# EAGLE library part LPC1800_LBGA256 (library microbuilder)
Generic LPC1800 LBGA256 Package
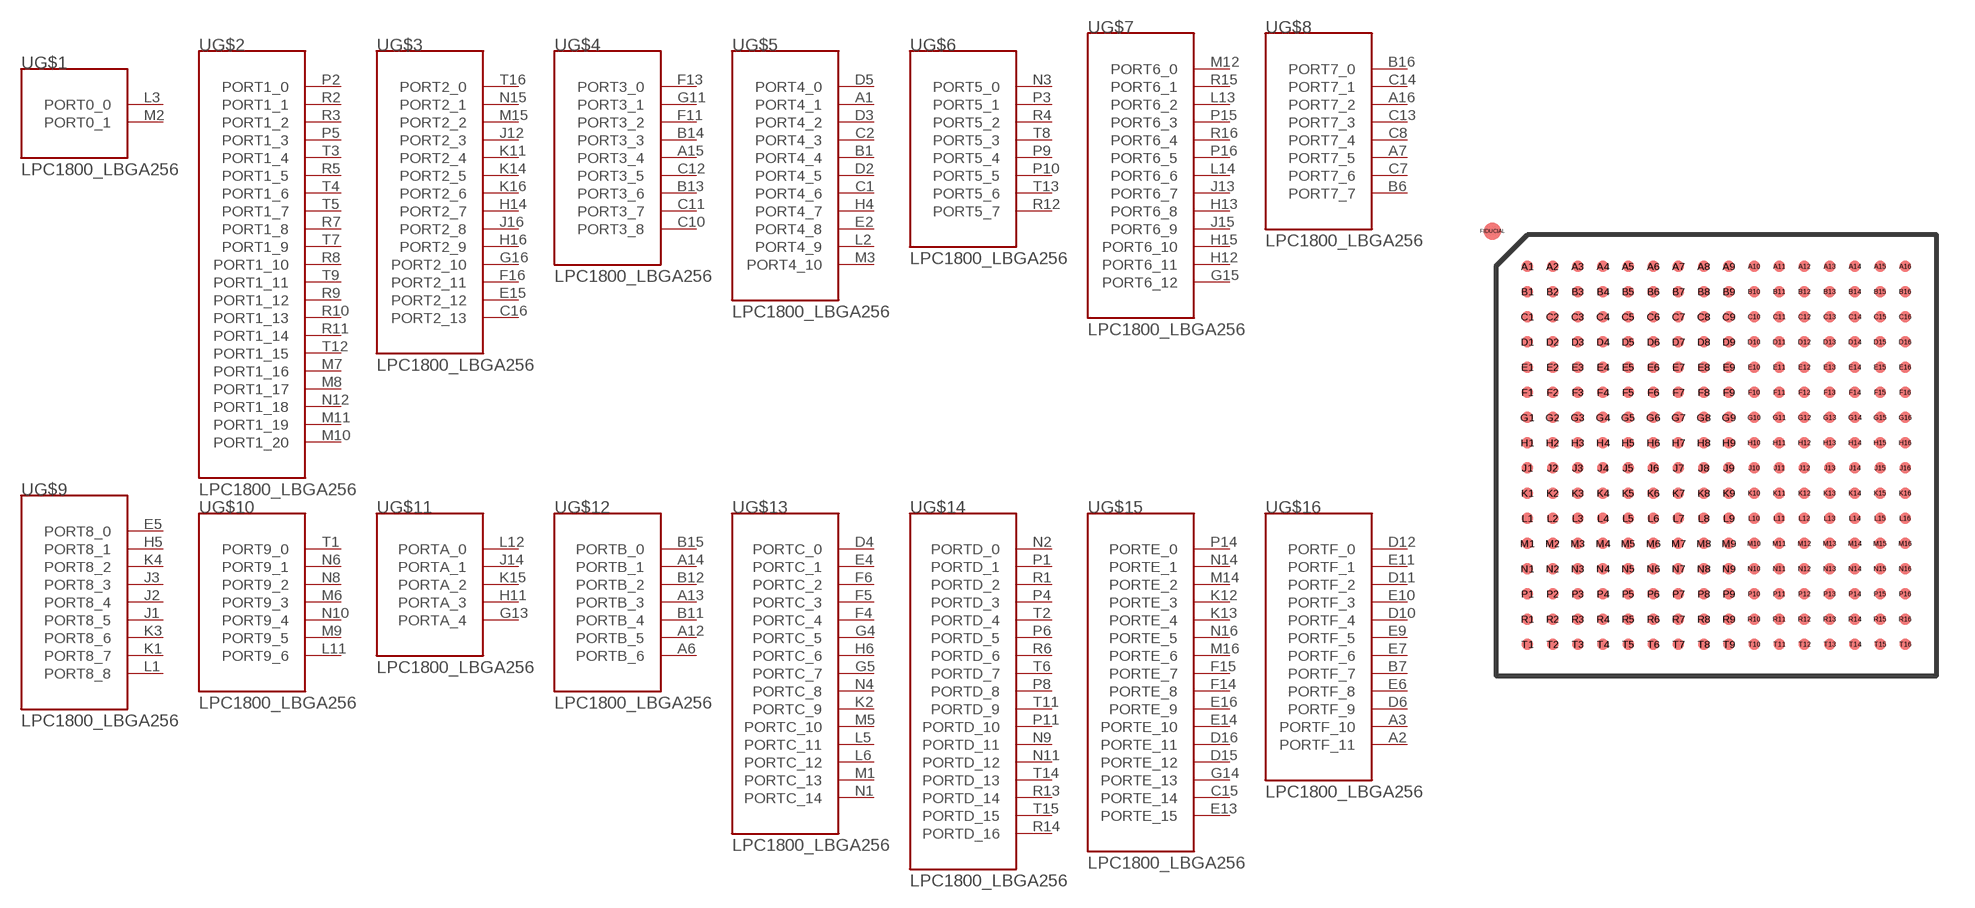
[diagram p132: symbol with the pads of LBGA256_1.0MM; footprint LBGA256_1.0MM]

Designator prefix U; gates G$1=LPC1800_PORT0 G$2=LPC1800_PORT1 G$3=LPC1800_PORT2 G$4=LPC1800_PORT3 G$5=LPC1800_PORT4 G$6=LPC1800_PORT5 G$7=LPC1800_PORT6 G$8=LPC1800_PORT7 G$9=LPC1800_PORT8 G$10=LPC1800_PORT9 G$11=LPC1800_PORTA G$12=LPC1800_PORTB G$13=LPC1800_PORTC G$14=LPC1800_PORTD G$15=LPC1800_PORTE G$16=LPC1800_PORTF G$17=LPC1800_ANA G$18=LPC1800_AO G$19=LPC1800_CLK G$20=LPC1800_DBUG G$21=LPC1800_SUP G$22=LPC1800_USB G$23=LPC1800_I2C

## LPC1800_LBGA256  [LBGA256_1.0MM]
A1  G$5:PORT4_1
A2  G$16:PORTF_11
A3  G$16:PORTF_10
A4  G$17:ADC2
A5  G$17:ADC6
A6  G$12:PORTB_6
A7  G$8:PORT7_5
A8  G$18:RTCX1
A9  G$18:WAKEUP0
A10  G$18:WAKEUP1
A11  G$18:ALARM
A12  G$12:PORTB_5
A13  G$12:PORTB_3
A14  G$12:PORTB_1
A15  G$4:PORT3_4
A16  G$8:PORT7_2
B1  G$5:PORT4_4
B2  G$17:VSSA  sup
B3  G$17:ADC5
B4  G$17:VDDA  sup
B5  G$17:ADC3
B6  G$8:PORT7_7
B7  G$16:PORTF_7
B8  G$18:RTXC2
B9  G$18:SAMPLE_N
B10  G$18:VBAT
B11  G$12:PORTB_4
B12  G$12:PORTB_2
B13  G$4:PORT3_6
B14  G$4:PORT3_3
B15  G$12:PORTB_0
B16  G$8:PORT7_0
C1  G$5:PORT4_6
C2  G$5:PORT4_3
C3  G$17:ADC1
C4  G$21:VSS  sup
C5  G$17:ADC7
C6  G$17:ADC4
C7  G$8:PORT7_6
C8  G$8:PORT7_4
C9  G$18:WAKEUP2
C10  G$4:PORT3_8
C11  G$4:PORT3_7
C12  G$4:PORT3_5
C13  G$8:PORT7_3
C14  G$8:PORT7_1
C15  G$15:PORTE_14
C16  G$3:PORT2_13
D1  G$19:XTAL1
D2  G$5:PORT4_5
D3  G$5:PORT4_2
D4  G$13:PORTC_0
D5  G$5:PORT4_0
D6  G$16:PORTF_9
D7  G$21:VDDE  sup
D8  G$18:WAKEUP3
D9  G$18:RESET
D10  G$16:PORTF_4
D11  G$16:PORTF_2
D12  G$16:PORTF_0
D13  G$21:VSS  sup
D14  G$19:CLK2
D15  G$15:PORTE_12
D16  G$15:PORTE_11
E1  G$19:XTAL2
E2  G$5:PORT4_8
E3  G$17:ADC0
E4  G$13:PORTC_1
E5  G$9:PORT8_0
E6  G$16:PORTF_8
E7  G$16:PORTF_6
E8  G$21:VPP  sup
E9  G$16:PORTF_5
E10  G$16:PORTF_3
E11  G$16:PORTF_1
E12  G$21:VDDE  sup
E13  G$15:PORTE_15
E14  G$15:PORTE_10
E15  G$3:PORT2_12
E16  G$15:PORTE_9
F1  G$22:USB_VBUS
F2  G$22:USB_DP0
F3  G$22:USB_VDDA3V3_DRIVER
F4  G$13:PORTC_4
F5  G$13:PORTC_3
F6  G$13:PORTC_2
F7  G$21:VDDE  sup
F8  G$21:VDDE  sup
F9  G$21:VDDC  sup
F10  G$21:VDDC  sup
F11  G$4:PORT3_2
F12  G$22:USB_DP1
F13  G$4:PORT3_0
F14  G$15:PORTE_8
F15  G$15:PORTE_7
F16  G$3:PORT2_11
G1  G$22:USB_VSSA_REF
G2  G$22:USB_DM0
G3  G$22:USB_VDDA3V3
G4  G$13:PORTC_5
G5  G$13:PORTC_7
G6  G$21:VSS  sup
G7  G$21:VSS  sup
G8  G$21:VSS  sup
G9  G$21:VSS  sup
G10  G$21:VDDE  sup
G11  G$4:PORT3_1
G12  G$22:USB_DM1
G13  G$11:PORTA_4
G14  G$15:PORTE_13
G15  G$7:PORT6_12
G16  G$3:PORT2_10
H1  G$22:USB_RREF
H2  G$22:USB_ID
H3  G$22:USB_VSSA_TERM
H4  G$5:PORT4_7
H5  G$9:PORT8_1
H6  G$13:PORTC_6
H7  G$21:VSS  sup
H8  G$21:VSS  sup
H9  G$21:VSS  sup
H10  G$21:VDDE  sup
H11  G$11:PORTA_3
H12  G$7:PORT6_11
H13  G$7:PORT6_8
H14  G$3:PORT2_7
H15  G$7:PORT6_10
H16  G$3:PORT2_9
J1  G$9:PORT8_5
J2  G$9:PORT8_4
J3  G$9:PORT8_3
J4  G$20:TDI
J5  G$20:TCK
J6  G$21:VDDE  sup
J7  G$21:VDDE  sup
J8  G$21:VSS  sup
J9  G$21:VSS  sup
J10  G$21:VSS  sup
J11  G$21:VSS  sup
J12  G$3:PORT2_3
J13  G$7:PORT6_7
J14  G$11:PORTA_1
J15  G$7:PORT6_9
J16  G$3:PORT2_8
K1  G$9:PORT8_7
K2  G$13:PORTC_9
K3  G$9:PORT8_6
K4  G$9:PORT8_2
K5  G$20:TDO
K6  G$20:TMS
K7  G$21:VDDE  sup
K8  G$21:VSS  sup
K9  G$21:VSS  sup
K10  G$21:VSS  sup
K11  G$3:PORT2_4
K12  G$15:PORTE_3
K13  G$15:PORTE_4
K14  G$3:PORT2_5
K15  G$11:PORTA_2
K16  G$3:PORT2_6
L1  G$9:PORT8_8  sup
L2  G$5:PORT4_9
L3  G$1:PORT0_0
L4  G$20:DBGEN
L5  G$13:PORTC_11
L6  G$13:PORTC_12
L7  G$21:VDDC  sup
L8  G$21:VDDC  sup
L9  G$21:VDDE  sup
L10  G$21:VDDE  sup
L11  G$10:PORT9_6
L12  G$11:PORTA_0
L13  G$7:PORT6_2
L14  G$7:PORT6_6
L15  G$23:SCL  sup
L16  G$23:SDA  sup
M1  G$13:PORTC_13
M2  G$1:PORT0_1
M3  G$5:PORT4_10
M4  G$20:TRST
M5  G$13:PORTC_10
M6  G$10:PORT9_3
M7  G$2:PORT1_16
M8  G$2:PORT1_17
M9  G$10:PORT9_5
M10  G$2:PORT1_20
M11  G$2:PORT1_19
M12  G$7:PORT6_0
M13  G$21:VSS  sup
M14  G$15:PORTE_2
M15  G$3:PORT2_2
M16  G$15:PORTE_6
N1  G$13:PORTC_14
N2  G$14:PORTD_0
N3  G$6:PORT5_0
N4  G$13:PORTC_8
N5  G$19:CLK0
N6  G$10:PORT9_1
N7  G$21:VDDE  sup
N8  G$10:PORT9_2
N9  G$14:PORTD_11
N10  G$10:PORT9_4
N11  G$14:PORTD_12
N12  G$2:PORT1_18
N13  G$21:VDDE  sup
N14  G$15:PORTE_1
N15  G$3:PORT2_1
N16  G$15:PORTE_5
P1  G$14:PORTD_1
P2  G$2:PORT1_0
P3  G$6:PORT5_1
P4  G$14:PORTD_3
P5  G$2:PORT1_3
P6  G$14:PORTD_5
P7  G$21:VSS  sup
P8  G$14:PORTD_8
P9  G$6:PORT5_4
P10  G$6:PORT5_5
P11  G$14:PORTD_10
P12  G$19:CLK3
P13  G$21:VSS  sup
P14  G$15:PORTE_0
P15  G$7:PORT6_3
P16  G$7:PORT6_5
R1  G$14:PORTD_2
R2  G$2:PORT1_1
R3  G$2:PORT1_2
R4  G$6:PORT5_2
R5  G$2:PORT1_5
R6  G$14:PORTD_6
R7  G$2:PORT1_8
R8  G$2:PORT1_10
R9  G$2:PORT1_12
R10  G$2:PORT1_13
R11  G$2:PORT1_14
R12  G$6:PORT5_7
R13  G$14:PORTD_14
R14  G$14:PORTD_16
R15  G$7:PORT6_1
R16  G$7:PORT6_4
T1  G$10:PORT9_0
T2  G$14:PORTD_4
T3  G$2:PORT1_4
T4  G$2:PORT1_6
T5  G$2:PORT1_7
T6  G$14:PORTD_7
T7  G$2:PORT1_9
T8  G$6:PORT5_3
T9  G$2:PORT1_11
T10  G$19:CLK1
T11  G$14:PORTD_9
T12  G$2:PORT1_15
T13  G$6:PORT5_6
T14  G$14:PORTD_13
T15  G$14:PORTD_15
T16  G$3:PORT2_0

## Footprint LBGA256_1.0MM (pad centres in mm)
LBGA256 - SOT740-2 LBGA256: plastic low profile ball grid array package; 256 balls; body 17 x 17 x 1 mm
smd 0.45 x 0.45: A1 -7.5,7.5; A2 -6.5,7.5; A3 -5.5,7.5; A4 -4.5,7.5; A5 -3.5,7.5; A6 -2.5,7.5; A7 -1.5,7.5; A8 -0.5,7.5; A9 0.5,7.5; A10 1.5,7.5; A11 2.5,7.5; A12 3.5,7.5; A13 4.5,7.5; A14 5.5,7.5; A15 6.5,7.5; A16 7.5,7.5; B1 -7.5,6.5; B2 -6.5,6.5; B3 -5.5,6.5; B4 -4.5,6.5; B5 -3.5,6.5; B6 -2.5,6.5; B7 -1.5,6.5; B8 -0.5,6.5; B9 0.5,6.5; B10 1.5,6.5; B11 2.5,6.5; B12 3.5,6.5; B13 4.5,6.5; B14 5.5,6.5; B15 6.5,6.5; B16 7.5,6.5; C1 -7.5,5.5; C2 -6.5,5.5; C3 -5.5,5.5; C4 -4.5,5.5; C5 -3.5,5.5; C6 -2.5,5.5; C7 -1.5,5.5; C8 -0.5,5.5; C9 0.5,5.5; C10 1.5,5.5; C11 2.5,5.5; C12 3.5,5.5; C13 4.5,5.5; C14 5.5,5.5; C15 6.5,5.5; C16 7.5,5.5; D1 -7.5,4.5; D2 -6.5,4.5; D3 -5.5,4.5; D4 -4.5,4.5; D5 -3.5,4.5; D6 -2.5,4.5; D7 -1.5,4.5; D8 -0.5,4.5; D9 0.5,4.5; D10 1.5,4.5; D11 2.5,4.5; D12 3.5,4.5; D13 4.5,4.5; D14 5.5,4.5; D15 6.5,4.5; D16 7.5,4.5; E1 -7.5,3.5; E2 -6.5,3.5; E3 -5.5,3.5; E4 -4.5,3.5; E5 -3.5,3.5; E6 -2.5,3.5; E7 -1.5,3.5; E8 -0.5,3.5; E9 0.5,3.5; E10 1.5,3.5; E11 2.5,3.5; E12 3.5,3.5; E13 4.5,3.5; E14 5.5,3.5; E15 6.5,3.5; E16 7.5,3.5; F1 -7.5,2.5; F2 -6.5,2.5; F3 -5.5,2.5; F4 -4.5,2.5; F5 -3.5,2.5; F6 -2.5,2.5; F7 -1.5,2.5; F8 -0.5,2.5; F9 0.5,2.5; F10 1.5,2.5; F11 2.5,2.5; F12 3.5,2.5; F13 4.5,2.5; F14 5.5,2.5; F15 6.5,2.5; F16 7.5,2.5; G1 -7.5,1.5; G2 -6.5,1.5; G3 -5.5,1.5; G4 -4.5,1.5; G5 -3.5,1.5; G6 -2.5,1.5; G7 -1.5,1.5; G8 -0.5,1.5; G9 0.5,1.5; G10 1.5,1.5; G11 2.5,1.5; G12 3.5,1.5; G13 4.5,1.5; G14 5.5,1.5; G15 6.5,1.5; G16 7.5,1.5; H1 -7.5,0.5; H2 -6.5,0.5; H3 -5.5,0.5; H4 -4.5,0.5; H5 -3.5,0.5; H6 -2.5,0.5; H7 -1.5,0.5; H8 -0.5,0.5; H9 0.5,0.5; H10 1.5,0.5; H11 2.5,0.5; H12 3.5,0.5; H13 4.5,0.5; H14 5.5,0.5; H15 6.5,0.5; H16 7.5,0.5; J1 -7.5,-0.5; J2 -6.5,-0.5; J3 -5.5,-0.5; J4 -4.5,-0.5; J5 -3.5,-0.5; J6 -2.5,-0.5; J7 -1.5,-0.5; J8 -0.5,-0.5; J9 0.5,-0.5; J10 1.5,-0.5; J11 2.5,-0.5; J12 3.5,-0.5; J13 4.5,-0.5; J14 5.5,-0.5; J15 6.5,-0.5; J16 7.5,-0.5; K1 -7.5,-1.5; K2 -6.5,-1.5; K3 -5.5,-1.5; K4 -4.5,-1.5; K5 -3.5,-1.5; K6 -2.5,-1.5; K7 -1.5,-1.5; K8 -0.5,-1.5; K9 0.5,-1.5; K10 1.5,-1.5; K11 2.5,-1.5; K12 3.5,-1.5; K13 4.5,-1.5; K14 5.5,-1.5; K15 6.5,-1.5; K16 7.5,-1.5; L1 -7.5,-2.5; L2 -6.5,-2.5; L3 -5.5,-2.5; L4 -4.5,-2.5; L5 -3.5,-2.5; L6 -2.5,-2.5; L7 -1.5,-2.5; L8 -0.5,-2.5; L9 0.5,-2.5; L10 1.5,-2.5; L11 2.5,-2.5; L12 3.5,-2.5; L13 4.5,-2.5; L14 5.5,-2.5; L15 6.5,-2.5; L16 7.5,-2.5; M1 -7.5,-3.5; M2 -6.5,-3.5; M3 -5.5,-3.5; M4 -4.5,-3.5; M5 -3.5,-3.5; M6 -2.5,-3.5; M7 -1.5,-3.5; M8 -0.5,-3.5; M9 0.5,-3.5; M10 1.5,-3.5; M11 2.5,-3.5; M12 3.5,-3.5; M13 4.5,-3.5; M14 5.5,-3.5; M15 6.5,-3.5; M16 7.5,-3.5; N1 -7.5,-4.5; N2 -6.5,-4.5; N3 -5.5,-4.5; N4 -4.5,-4.5; N5 -3.5,-4.5; N6 -2.5,-4.5; N7 -1.5,-4.5; N8 -0.5,-4.5; N9 0.5,-4.5; N10 1.5,-4.5; N11 2.5,-4.5; N12 3.5,-4.5; N13 4.5,-4.5; N14 5.5,-4.5; N15 6.5,-4.5; N16 7.5,-4.5; P1 -7.5,-5.5; P2 -6.5,-5.5; P3 -5.5,-5.5; P4 -4.5,-5.5; P5 -3.5,-5.5; P6 -2.5,-5.5; P7 -1.5,-5.5; P8 -0.5,-5.5; P9 0.5,-5.5; P10 1.5,-5.5; P11 2.5,-5.5; P12 3.5,-5.5; P13 4.5,-5.5; P14 5.5,-5.5; P15 6.5,-5.5; P16 7.5,-5.5; R1 -7.5,-6.5; R2 -6.5,-6.5; R3 -5.5,-6.5; R4 -4.5,-6.5; R5 -3.5,-6.5; R6 -2.5,-6.5; R7 -1.5,-6.5; R8 -0.5,-6.5; R9 0.5,-6.5; R10 1.5,-6.5; R11 2.5,-6.5; R12 3.5,-6.5; R13 4.5,-6.5; R14 5.5,-6.5; R15 6.5,-6.5; R16 7.5,-6.5; T1 -7.5,-7.5; T2 -6.5,-7.5; T3 -5.5,-7.5; T4 -4.5,-7.5; T5 -3.5,-7.5; T6 -2.5,-7.5; T7 -1.5,-7.5; T8 -0.5,-7.5; T9 0.5,-7.5; T10 1.5,-7.5; T11 2.5,-7.5; T12 3.5,-7.5; T13 4.5,-7.5; T14 5.5,-7.5; T15 6.5,-7.5; T16 7.5,-7.5
smd 0.7 x 0.7: FIDUCIAL -8.89,8.89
